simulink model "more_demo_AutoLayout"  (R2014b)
settings: Solver=ode45  StartTime=0.0  StopTime=10.0  RelTol=1e-3
libraries: simulink x2

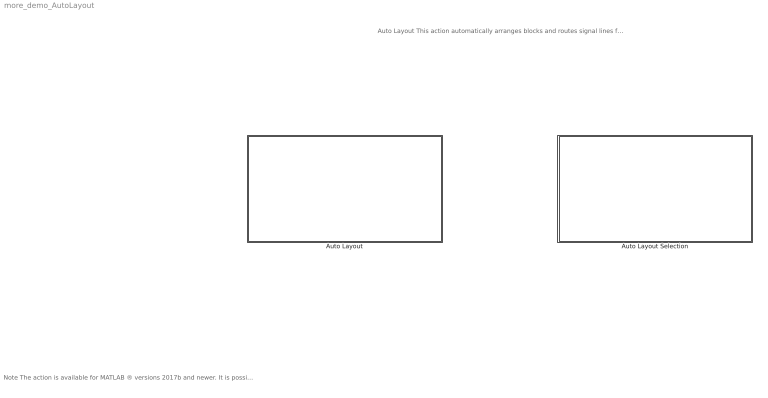
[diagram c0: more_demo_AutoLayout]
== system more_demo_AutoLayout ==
  note: Note The action is available for MATLAB ® versions 2017b and newer. It is possible to set custom parameters for blocks and lines with this action. Simply activate the feature via "Preferences -> Config File" and set "ApplyMoRePreferencesToBlocksAndLines" to true. In some cases, you may not want blocks without ports to be repositioned when applying the "Auto Layout" action. You can use a configuration parameter to exclude such blocks from the action. Simply activate the feature via "Preferences -> Config File" and set "IncludeBlocksWithoutPorts" to false.
  note: Auto Layout This action automatically arranges blocks and routes signal lines for a clean and uniform layout. This action can be applied to an entire subsystem or a selection of blocks. Navigate to the respective subsystem for a corresponding demonstration.
  Auto Layout : Subsystem
  Auto Layout Selection : Subsystem

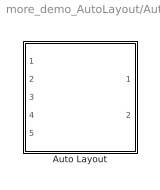
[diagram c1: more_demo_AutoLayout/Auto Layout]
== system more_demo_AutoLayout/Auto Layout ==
  Auto Layout : Subsystem

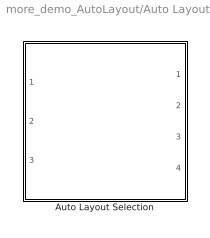
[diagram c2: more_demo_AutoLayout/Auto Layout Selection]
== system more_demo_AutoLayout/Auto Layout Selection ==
  Auto Layout Selection : Subsystem

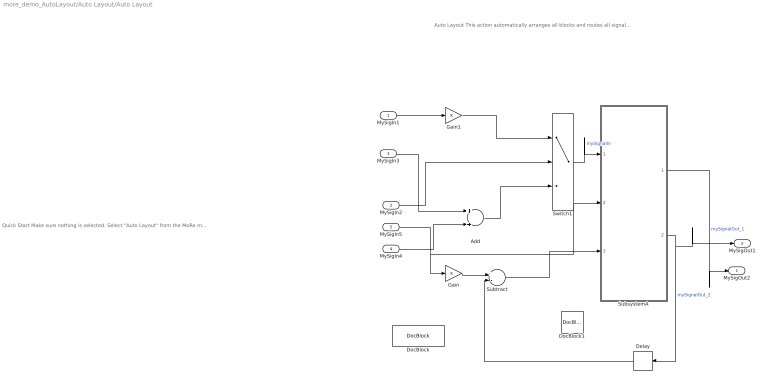
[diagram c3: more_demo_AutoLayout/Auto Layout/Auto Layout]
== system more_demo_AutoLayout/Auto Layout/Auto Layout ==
  note: Quick Start Make sure nothing is selected. Select "Auto Layout" from the MoRe menu and note the changes.
  note: Auto Layout This action automatically arranges all blocks and routes all signal lines in the current subsystem for a clean and uniform layout.
  MySigIn1 : Inport
  MySigIn2 : Inport  Port=2
  MySigIn3 : Inport  Port=3
  MySigIn4 : Inport  Port=4
  MySigIn5 : Inport  Port=5
  Add : Sum
  Delay : Delay
  DocBlock : simulink/Model-Wide Utilities/DocBlock  DocumentType=Text
  DocBlock1 : simulink/Model-Wide Utilities/DocBlock  DocumentType=Text
  Gain : Gain
  Gain1 : Gain
  SubsystemA : Subsystem
  Subtract : Sum  Inputs=+-
  Switch1 : Switch  Criteria=u2 > Threshold
  MySigOut2 : Outport
  MySigOut1 : Outport  Port=2
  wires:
  MySigIn4/1 -> Add/2
  MySigIn3/1 -> Add/1
  Add/1 -> Switch1/3
  MySigIn1/1 -> Gain1/1
  Gain1/1 -> Switch1/1
  MySigIn2/1 -> Switch1/2
  Switch1/1 -> SubsystemA/1(MySig1)  "mySignalIn"
  MySigIn5/1 -> Gain/1, SubsystemA/2(MySig2)
  Gain/1 -> Subtract/1
  SubsystemA/2(Result2) -> MySigOut1/1, Delay/1  "mySignalOut_2"
  Delay/1 -> Subtract/2
  Subtract/1 -> SubsystemA/3(MySig3)
  SubsystemA/1(Result1) -> MySigOut2/1  "mySignalOut_1"

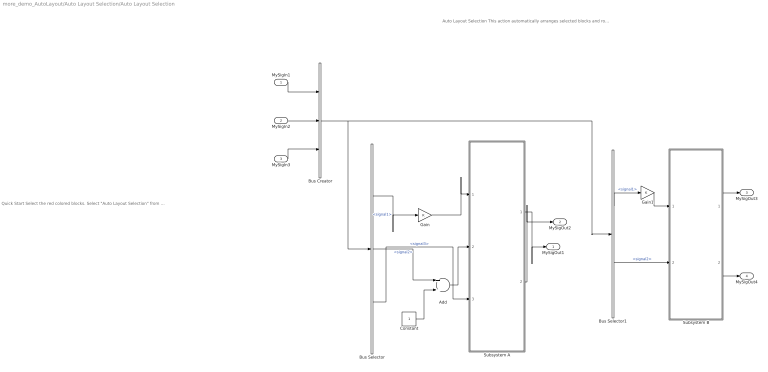
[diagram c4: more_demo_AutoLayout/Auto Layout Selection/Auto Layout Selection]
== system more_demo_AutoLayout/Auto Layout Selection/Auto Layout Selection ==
  note: Quick Start Select the red colored blocks. Select "Auto Layout Selection" from the MoRe menu and note the changes.
  note: Auto Layout Selection This action automatically arranges selected blocks and routes the signal lines connected to these blocks for a clean and uniform layout.
  MySigIn1 : Inport
  MySigIn2 : Inport  Port=2
  MySigIn3 : Inport  Port=3
  Add : Sum
  Bus Creator : BusCreator  Inputs=3
  Bus Selector : BusSelector
  Bus Selector1 : BusSelector  OutputSignals=signal1,signal2
  Constant : Constant
  Gain : Gain
  Gain1 : Gain
  Subsystem A : Subsystem
  Subsystem B : Subsystem
  MySigOut1 : Outport
  MySigOut2 : Outport  Port=2
  MySigOut3 : Outport  Port=3
  MySigOut4 : Outport  Port=4
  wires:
  Bus Creator/1 -> Bus Selector1/1, Bus Selector/1
  Constant/1 -> Add/2
  Bus Selector/2 -> Add/1  "<signal2>"
  Add/1 -> Subsystem A/2("MySig2 ")
  Bus Selector/1 -> Gain/1  "<signal1>"
  Gain/1 -> Subsystem A/1(MySig1)
  Subsystem A/1(Result1) -> MySigOut1/1
  Subsystem A/2(Result2) -> MySigOut2/1
  Bus Selector1/2 -> Subsystem B/2("MySig2 ")  "<signal2>"
  Bus Selector1/1 -> Gain1/1  "<signal1>"
  Gain1/1 -> Subsystem B/1(MySig1)
  Subsystem B/1(Result1) -> MySigOut3/1
  Subsystem B/2(Result2) -> MySigOut4/1
  MySigIn1/1 -> Bus Creator/1
  MySigIn2/1 -> Bus Creator/2
  MySigIn3/1 -> Bus Creator/3
  Bus Selector/3 -> Subsystem A/3(MySig3)  "<signal3>"

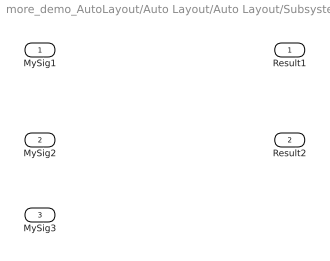
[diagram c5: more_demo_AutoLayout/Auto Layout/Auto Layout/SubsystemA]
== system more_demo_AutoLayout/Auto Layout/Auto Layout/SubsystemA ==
  MySig1 : Inport
  MySig2 : Inport  Port=2
  MySig3 : Inport  Port=3
  Result1 : Outport
  Result2 : Outport  Port=2

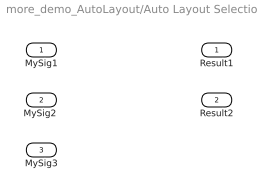
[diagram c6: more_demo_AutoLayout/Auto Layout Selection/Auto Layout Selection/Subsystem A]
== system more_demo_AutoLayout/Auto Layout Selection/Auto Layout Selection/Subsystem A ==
  MySig1 : Inport
  "MySig2 " : Inport  Port=2
  MySig3 : Inport  Port=3
  Result1 : Outport
  Result2 : Outport  Port=2

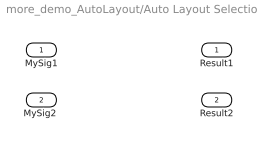
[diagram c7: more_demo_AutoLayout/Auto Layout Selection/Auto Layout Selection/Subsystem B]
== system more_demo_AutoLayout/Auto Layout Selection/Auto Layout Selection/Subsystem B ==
  MySig1 : Inport
  "MySig2 " : Inport  Port=2
  Result1 : Outport
  Result2 : Outport  Port=2
